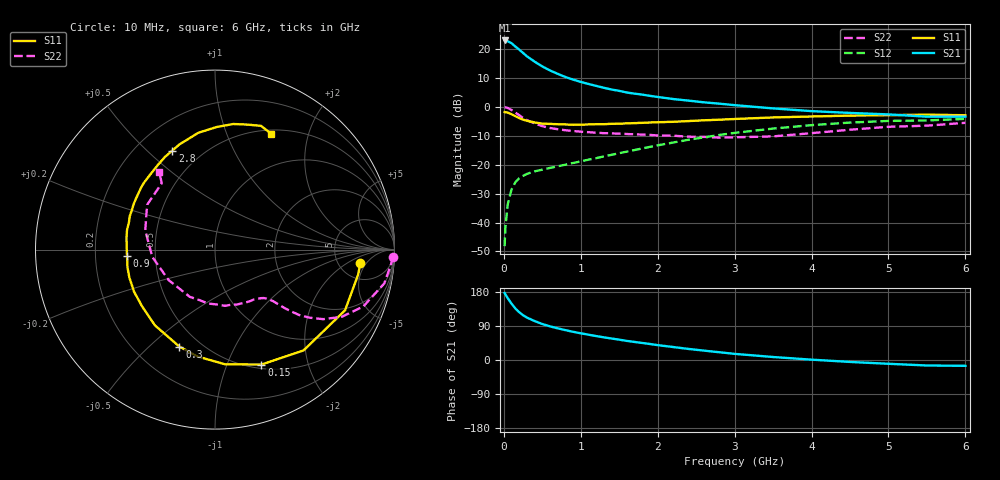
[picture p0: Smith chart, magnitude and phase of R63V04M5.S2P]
! SIEMENS Small Signal Semiconductors
! BFR193
! Si NPN RF Bipolar Junction Transistor in SOT23
! VCE = 3 V  IC = 4.5 mA
! Common Emitter S-Parameters:  May  1996
# GHz  S  MA  R  50
!  f  S11  S21  S12  S22
! GHz  MAG  ANG  MAG  ANG  MAG  ANG  MAG  ANG
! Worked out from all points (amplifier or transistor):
!   36 points, 10 MHz to 6 GHz, reference 50 ohm
!   highest |S21| = 23.0 dB at 10 MHz (marker M1)
!   |S21| within 3 dB of that: start of sweep to 192.5 MHz
!   unconditionally stable (mu >= 1): 922.1 MHz to 1.971 GHz
!   at 250 MHz: K = 0.40, MSG = 21.3 dB, |S12| = -23.8 dB
!   at 1.4 GHz: K = 1.07, MAG = 9.7 dB, |S12| = -16.6 dB
!   at 6 GHz: K = 0.97, MSG = 0.4 dB, |S12| = -4.1 dB
!   S11 on the Smith chart (normalised r, x): 10 MHz: 8.12, -3.62; 150 MHz: 0.54, -1.33; 300 MHz: 0.39, -0.62; 900 MHz: 0.34, -0.03; 2.8 GHz: 0.35, +0.60; 6 GHz: 0.54, +1.45
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0.01  0.8141 -5.3  14.12 176.8  0.0039 89.6  0.9921 -2.3
0.02  0.8094 -10.0  13.86 173.1  0.0082 82.4  0.9849 -4.6
0.05  0.7996 -25.0  13.69 163.4  0.0205 77.3  0.9619 -11.3
0.1  0.7476 -48.7  12.64 148.6  0.0374 66.8  0.8849 -21.0
0.15  0.6907 -68.0  11.06 135.8  0.0499 58.8  0.7999 -27.9
0.2  0.6414 -85.0  9.819 126.1  0.0585 53.3  0.7175 -32.7
0.25  0.6037 -99.2  8.582 118.0  0.0642 49.5  0.646 -35.9
0.3  0.5755 -110.2  7.517 112.0  0.0694 47.7  0.5922 -37.9
0.4  0.5387 -128.4  6.074 102.8  0.0768 45.2  0.5179 -39.8
0.5  0.5147 -142.2  5.013 94.9  0.0821 45.6  0.4644 -40.9
0.6  0.5083 -152.6  4.279 88.8  0.0881 46.7  0.4321 -41.6
0.7  0.5019 -161.8  3.736 83.5  0.094 48.1  0.4113 -42.6
0.9  0.4912 -176.0  2.972 74.4  0.1072 51.1  0.3831 -44.8
1.1  0.4978 172.1  2.496 66.8  0.1224 54.3  0.3652 -48.5
1.3  0.5023 163.0  2.144 59.8  0.1396 56.7  0.3517 -52.4
1.6  0.5194 150.8  1.774 50.3  0.1688 58.5  0.34 -60.2
2.2  0.5527 130.6  1.369 34.3  0.2419 57.5  0.3181 -79.9
2.8  0.6006 113.3  1.139 20.5  0.3269 51.5  0.2945 -107.4
3.5  0.6576 98.1  0.943 7.9  0.4222 40.9  0.3093 -146.6
4.5  0.7073 81.7  0.787 -5.1  0.536 23.5  0.4031 164.6
5.5  0.7356 69.6  0.678 -14.5  0.5838 6.2  0.4738 128.8
6  0.7177 64.2  0.679 -15.4  0.6206 1.2  0.5311 125.7
